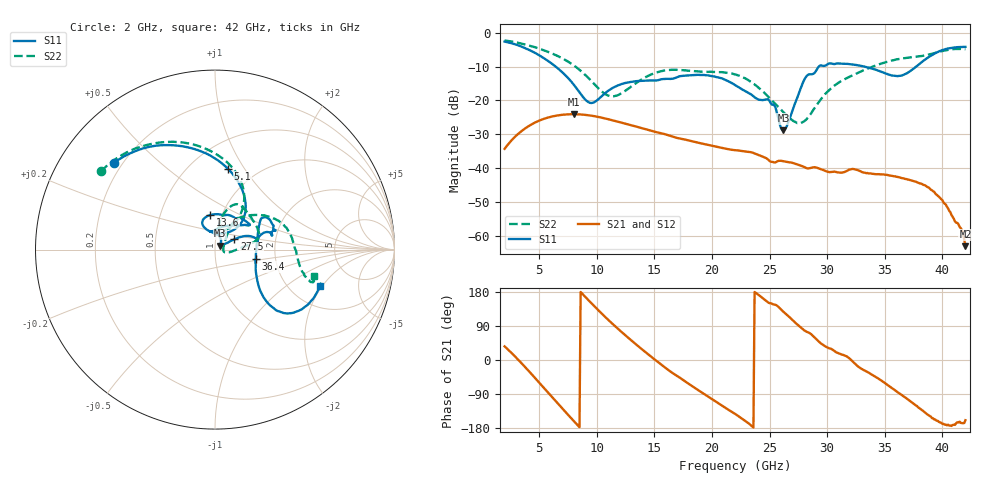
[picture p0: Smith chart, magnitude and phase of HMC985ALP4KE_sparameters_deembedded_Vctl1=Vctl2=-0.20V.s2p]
!s2p File: Measurements: S11, S21, S12, S22
# GHz S dB R 50.0
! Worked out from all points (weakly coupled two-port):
!   401 points, 2 GHz to 42 GHz, reference 50 ohm
!   highest |S21| = -24.05 dB at 8 GHz (marker M1); lowest = -63.0 dB at 42 GHz (marker M2)
!   lowest |S11| = -28.9 dB at 26.2 GHz (marker M3), VSWR 1.07, Z = 52.9 + j2.33 ohm
!   |S11| at or under -10 dB: 6.437 GHz to 29.27 GHz (22.84 GHz wide, 128 % of centre); 33.25 GHz to 37.73 GHz (4.475 GHz wide, 12.6 % of centre)
!   |S22| runs from -26.7 to -2.3 dB; largest |S21 - S12| = 0.00016
!   S11 on the Smith chart (normalised r, x): 2 GHz: 0.17, +0.36; 5.1 GHz: 0.75, +0.85; 13.6 GHz: 0.88, +0.35; 27.5 GHz: 1.23, +0.14; 36.4 GHz: 1.57, -0.17; 42 GHz: 2.92, -1.90
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2  -2.60 139.1  -34.29 36.0  -34.29 36.0  -2.26 145.6
3.5  -4.13 111.0  -28.97 -9.5  -28.98 -9.5  -3.22 121.8
5.1  -6.84 80.8  -25.82 -62.9  -25.83 -62.9  -4.79 97.4
8  -15.30 45.2  -24.05 -161.0  -24.06 -161.0  -9.61 60.5
8.7  -18.50 53.5  -24.15 176.3  -24.16 176.2  -11.51 55.5
9.6  -20.71 86.8  -24.52 147.8  -24.53 147.7  -14.48 53.4
11.2  -16.67 116.5  -25.72 100.1  -25.71 100.1  -18.73 68.9
13.6  -14.24 98.3  -27.88 36.3  -27.89 36.3  -14.43 77.9
15.4  -13.93 73.3  -29.51 -7.0  -29.52 -7.0  -11.50 68.3
19.4  -12.52 35.3  -32.93 -91.4  -32.94 -91.4  -11.51 34.4
22  -15.41 52.8  -34.69 -142.0  -34.68 -141.9  -12.29 13.7
25  -20.14 95.8  -37.87 150.0  -37.88 150.0  -19.29 -2.8
26.2  -28.86 37.7  -37.95 127.3  -37.97 127.3  -23.45 -14.6
27.5  -18.26 27.9  -39.00 91.6  -39.02 91.2  -26.64 -2.3
28.1  -13.33 20.0  -39.82 76.5  -39.83 76.3  -25.90 19.9
28.7  -12.24 12.2  -39.78 65.4  -39.84 65.4  -23.30 37.6
31.1  -9.12 23.5  -41.30 16.7  -41.30 16.3  -14.51 55.8
35.4  -12.39 12.1  -42.15 -69.3  -42.16 -69.3  -8.39 25.9
36.4  -12.69 -13.0  -42.85 -91.0  -42.86 -91.2  -7.62 17.2
39.9  -5.23 -40.4  -49.16 -165.7  -49.21 -165.8  -5.46 -17.0
41.6  -4.19 -21.7  -57.72 -166.0  -58.05 -166.4  -4.77 -17.4
42  -4.15 -18.9  -63.05 -159.0  -63.48 -160.3  -4.90 -14.8
